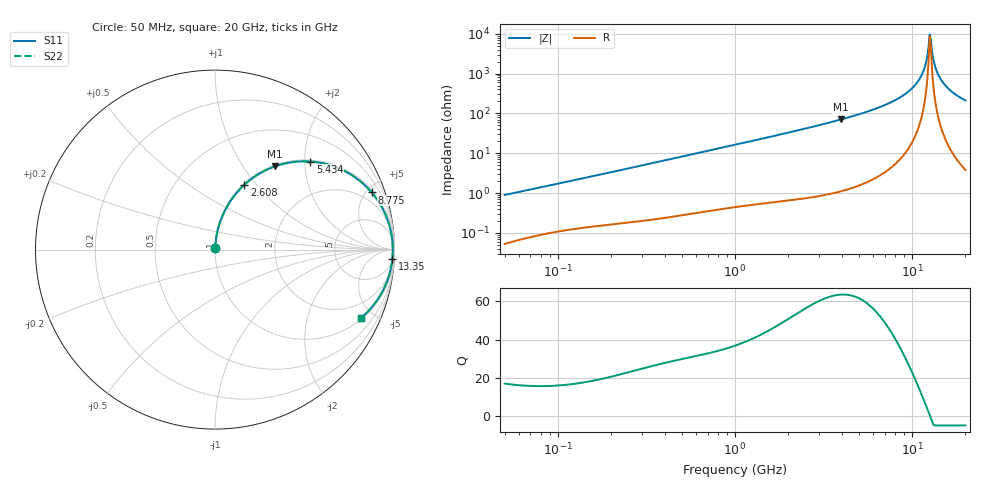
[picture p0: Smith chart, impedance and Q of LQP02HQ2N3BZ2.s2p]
!Murata Part Number: LQP02HQ2N3BZ2
!These Parameters are Measured in Series Mode Connection
!  o--[Z]--o
!Port1  Port2
!  o-------o
!Freq. Start=50[MHz] Stop=20[GHz], 401[Steps]
# Hz S RI R 50
!Freq.(Hz) S11(Real) S11(Imag) S21(Real) S21(Imag) S12(Real) S12(Imag) S22(Real) S22(Imag)
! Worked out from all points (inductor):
!   401 points, 50 MHz to 20 GHz, reference 50 ohm
!   read as one part in series: L = 2.81 nH near 51.52 MHz
!   highest Q = 63.5 at 3.967 GHz (marker M1), where L = 2.82 nH
!   self-resonance near 12.57 GHz
!   S11 on the Smith chart (normalised r, x): 50 MHz: 1.00, +0.02; 2.608 GHz: 1.02, +0.87; 5.434 GHz: 1.04, +2.13; 8.775 GHz: 1.16, +5.41; 13.35 GHz: 7, -35; 20 GHz: 1.08, -4.23
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5e7  0.000608 0.00893  0.9994 -0.00893  0.9994 -0.00893  0.000608 0.00893
1.364002e8  0.00186 0.023  0.9981 -0.023  0.9981 -0.023  0.00186 0.023
3.721004e8  0.006 0.0609  0.994 -0.0609  0.994 -0.0609  0.006 0.0609
1e9  0.0299 0.1574  0.9701 -0.1574  0.9701 -0.1574  0.0299 0.1574
2.608132e9  0.1642 0.3619  0.8358 -0.3619  0.8358 -0.3619  0.1642 0.3619
2.728004e9  0.1777 0.3738  0.8223 -0.3738  0.8223 -0.3738  0.1777 0.3738
3.967106e9  0.3336 0.4637  0.6664 -0.4637  0.6664 -0.4637  0.3336 0.4637
5.433528e9  0.531 0.4907  0.469 -0.4907  0.469 -0.4907  0.531 0.4907
7.442007e9  0.7633 0.4142  0.2367 -0.4142  0.2367 -0.4142  0.7633 0.4142
8.774992e9  0.8728 0.3187  0.1272 -0.3187  0.1272 -0.3187  0.8728 0.3187
1.004137e10  0.9414 0.2138  0.0586 -0.2138  0.0586 -0.2138  0.9414 0.2138
1.115139e10  0.9757 0.1196  0.0243 -0.1196  0.0243 -0.1196  0.9757 0.1196
1.183995e10  0.9866 0.0626  0.0134 -0.0626  0.0134 -0.0626  0.9866 0.0626
1.238412e10  0.9903 0.0191  0.00969 -0.0191  0.00969 -0.0191  0.9903 0.0191
1.257102e10  0.9907 0.00451  0.0093 -0.00451  0.0093 -0.00451  0.9907 0.00451
1.276073e10  0.9907 -0.0101  0.00934 0.0101  0.00934 0.0101  0.9907 -0.0101
1.295331e10  0.9902 -0.0246  0.0098 0.0246  0.0098 0.0246  0.9902 -0.0246
1.334722e10  0.988 -0.0537  0.012 0.0537  0.012 0.0537  0.988 -0.0537
1.417136e10  0.9784 -0.111  0.0216 0.111  0.0216 0.111  0.9784 -0.111
1.527346e10  0.9574 -0.18  0.0426 0.18  0.0426 0.18  0.9574 -0.18
1.721783e10  0.9047 -0.2801  0.0953 0.2801  0.0953 0.2801  0.9047 -0.2801
2e10  0.8133 -0.3808  0.1867 0.3808  0.1867 0.3808  0.8133 -0.3808
